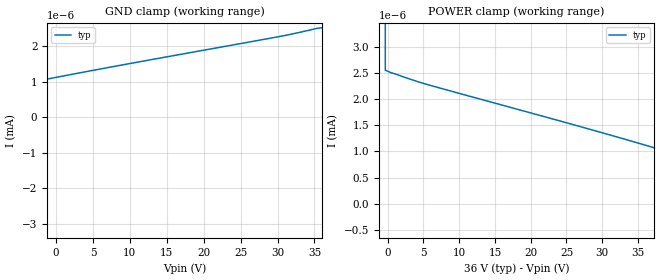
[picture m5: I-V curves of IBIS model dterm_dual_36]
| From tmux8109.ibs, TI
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| dterm_dual_36
[Model]   dterm_dual_36
Model_type   Terminator
|   typ   min   max
C_comp   4.014581e-12   NA   NA
[Voltage Range]   36   NA   NA
[Temperature Range]   27   NA   NA
[Power Clamp Reference]   36   NA   NA
[GND Clamp Reference]   0   NA   NA
[GND Clamp]
|   Voltage   I(typ)   I(min)   I(max)
-41V      -2.259A    NA         NA
-37.11V   -40.09mA   NA         NA
-36.33V   -3.132nA   NA         NA
-35.56V   -505.4pA   NA         NA
-30.89V   -313.9pA   NA         NA
-17.67V   352.5pA    NA         NA
-6.778V   841.9pA    NA         NA
6.444V    1.374nA    NA         NA
30.56V    2.284nA    NA         NA
36V       2.519nA    NA         NA
[POWER Clamp]
|   Voltage   I(typ)   I(min)   I(max)
-5V       744mA      NA         NA
-1.111V   26.13mA    NA         NA
-333.3mV  2.556nA    NA         NA
444.4mV   2.508nA    NA         NA
5.111V    2.297nA    NA         NA
29.22V    1.387nA    NA         NA
42.44V    856pA      NA         NA
53.33V    368.5pA    NA         NA
67.33V    -334.5pA   NA         NA
72V       -522.1pA   NA         NA
